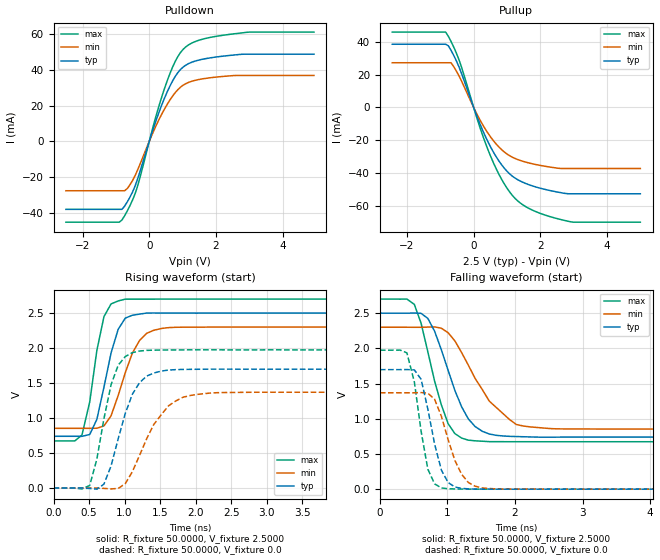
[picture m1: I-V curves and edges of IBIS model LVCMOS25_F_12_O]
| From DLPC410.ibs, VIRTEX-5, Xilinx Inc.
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|   Model LVCMOS25_F_12_O
[Model]  LVCMOS25_F_12_O
Model_type   Output
Polarity   Non-Inverting
Enable   Active-Low
Vmeas =  1.2500V
Cref =   0.0F
Rref =   1.0000M
Vref =   0.0V
C_comp   6.0000pF   6.0000pF   6.0000pF
[Model Spec]
[Temperature Range]   25.0000   85.0000   0.0
[Voltage Range]   2.5000V   2.3000V   2.7000V
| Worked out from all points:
|   slope of the pulldown table from 0 to 0.375 V, typ, clamps not added: 18.3 ohm
|   slope of the pullup table from 0 to 0.375 V, typ, clamps not added: 20 ohm
|   rising waveform, R_fixture 50.0000, V_fixture 2.5000: 20-80 % time 241ps typ, 308ps min, 203ps max; typ from 0.74 V to 2.5 V
|   rising waveform, R_fixture 50.0000, V_fixture 0.0: 20-80 % time 304ps typ, 428ps min, 242ps max; typ from 0 V to 1.7 V
|   falling waveform, R_fixture 50.0000, V_fixture 2.5000: 20-80 % time 409ps typ, 575ps min, 329ps max; typ from 2.5 V to 0.74 V
|   falling waveform, R_fixture 50.0000, V_fixture 0.0: 20-80 % time 234ps typ, 293ps min, 194ps max; typ from 1.7 V to 0 V
[Pulldown]
|Voltage   I(typ)   I(min)   I(max)
-2.5V     -38.19mA   -27.75mA   -45.4mA
-900mV    -38.19mA   -27.75mA   -45.4mA
-820mV    -38.19mA   -27.75mA   -44.17mA
-660mV    -34.01mA   -26.53mA   -39.08mA
-420mV    -24.85mA   -19.05mA   -29.15mA
140mV     8.212mA    6.157mA    9.988mA
540mV     27.82mA    20.82mA    34.08mA
860mV     38.63mA    29.04mA    47.66mA
1.1V      42.79mA    32.41mA    53.07mA
1.66V     46.29mA    35.24mA    57.61mA
2.7V      48.72mA    36.96mA    60.69mA
4.94V     48.9mA     36.96mA    61.3mA
[Pullup]
|Voltage   I(typ)   I(min)   I(max)
-2.44V    38.57mA    27.27mA    45.99mA
-840mV    38.57mA    27.27mA    45.99mA
-680mV    34.91mA    27.27mA    40.36mA
-600mV    31.85mA    24.98mA    36.97mA
-360mV    20.56mA    15.97mA    24.36mA
200mV     -10.61mA   -8.007mA   -12.92mA
600mV     -27.55mA   -20.5mA    -34.11mA
1V        -38.97mA   -28.46mA   -49.3mA
1.4V      -44.98mA   -32.4mA    -58.39mA
2.04V     -49.56mA   -35.57mA   -65.02mA
2.92V     -52.73mA   -37.31mA   -69.88mA
5V        -52.73mA   -37.31mA   -70.08mA
[Ramp]
dV/dt_r  1.0188/0.3043n   0.8214/0.4176n   1.1844/0.2422n
dV/dt_f  1.0563/0.4089n   0.8677/0.5655n   1.2158/0.3294n
R_load = 50.0000
[Rising Waveform]
R_fixture= 50.0000
V_fixture= 2.5000
V_fixture_min= 2.3000
V_fixture_max= 2.7000
|time   V(typ)   V(min)   V(max)
0s        739.5mV    853.9mV    673.7mV
400ps     739.4mV    853.9mV    757.5mV
510ps     765.5mV    853.9mV    1.233V
610ps     982.2mV    854.8mV    1.967V
710ps     1.442V     888.1mV    2.45V
910ps     2.268V     1.323V     2.673V
1.01ns    2.428V     1.649V     2.699V
1.21ns    2.485V     2.108V     2.699V
1.62ns    2.5V       2.292V     2.7V
10ns      2.5V       2.3V       2.7V
[Rising Waveform]
R_fixture= 50.0000
V_fixture= 0.0
|time   V(typ)   V(min)   V(max)
0s        3.489uV    4.276uV    3.426uV
510ps     -5.574mV   20.51uV    37.86mV
710ps     56.31mV    -4.636mV   993.8mV
810ps     317.4mV    -12.05mV   1.477V
910ps     704.8mV    -5.439mV   1.755V
1.11ns    1.342V     235.3mV    1.935V
1.21ns    1.505V     465.7mV    1.957V
1.62ns    1.686V     1.176V     1.973V
2.12ns    1.698V     1.349V     1.975V
10ns      1.698V     1.369V     1.974V
[Falling Waveform]
R_fixture= 50.0000
V_fixture= 2.5000
V_fixture_min= 2.3000
V_fixture_max= 2.7000
|time   V(typ)   V(min)   V(max)
0s        2.5V       2.3V       2.7V
510ps     2.502V     2.299V     2.624V
710ps     2.425V     2.302V     1.95V
810ps     2.244V     2.305V     1.535V
1.01ns    1.688V     2.222V     930.3mV
1.31ns    996.8mV    1.76V      695.7mV
1.62ns    783.6mV    1.25V      675mV
2.02ns    747.4mV    918.5mV    673.9mV
2.22ns    742mV      884.8mV    673.8mV
10ns      739.5mV    853.9mV    673.7mV
[Falling Waveform]
R_fixture= 50.0000
V_fixture= 0.0
|time   V(typ)   V(min)   V(max)
0s        1.698V     1.369V     1.974V
400ps     1.699V     1.369V     1.936V
510ps     1.694V     1.369V     1.524V
610ps     1.561V     1.372V     823.1mV
710ps     1.137V     1.363V     283.1mV
910ps     271.3mV    1.036V     17.21mV
1.01ns    94.47mV    703.7mV    6.569mV
1.21ns    11.34mV    211.4mV    1.286mV
1.52ns    780.8uV    16.8mV     186.3uV
10ns      2.694uV    4.14uV     3.208uV
